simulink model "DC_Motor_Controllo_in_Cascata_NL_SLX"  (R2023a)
settings: Solver=ode45  StartTime=0.0  StopTime=10.0  MaxStep=0.001  RelTol=1e-3
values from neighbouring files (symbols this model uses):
  b_m = 0.002*N/(m/sec)    (= 0.002)    [DC_Motor_Controllo_in_Cascata_NL_SLX_m.m]    (also in DC_Motor_Controllo_in_Cascata_SLX_m.m; Electrical_DC_Motor_EQN.m; Electrical_DC_Motor_SLX_m.m)
  C_p_0 = 0*Nm    (= 0)    [DC_Motor_Controllo_in_Cascata_NL_SLX_m.m]    (also in DC_Motor_Controllo_in_Cascata_SLX_m.m; Electrical_DC_Motor_SLX_m.m)
  I_a_0 = 0*A    (= 0)    [DC_Motor_Controllo_in_Cascata_NL_SLX_m.m]    (also in DC_Motor_Controllo_in_Cascata_SLX_m.m; Electrical_DC_Motor_SLX_m.m)
  J_m = 0.01*kg*m^2    (= 0.01)    [DC_Motor_Controllo_in_Cascata_NL_SLX_m.m]    (also in DC_Motor_Controllo_in_Cascata_SLX_m.m; Electrical_DC_Motor_EQN.m; Electrical_DC_Motor_SLX_m.m)
  K_I1 = 12532    [DC_Motor_Controllo_in_Cascata_NL_SLX_m.m]    (also in DC_Motor_Controllo_in_Cascata_SLX_m.m)
  K_m = 0.5    [DC_Motor_Controllo_in_Cascata_NL_SLX_m.m]    (also in DC_Motor_Controllo_in_Cascata_SLX_m.m; Electrical_DC_Motor_EQN.m; Electrical_DC_Motor_SLX_m.m)
  K_Thm = 100    [DC_Motor_Controllo_in_Cascata_NL_SLX_m.m]    (also in DC_Motor_Controllo_in_Cascata_SLX_m.m)
  K_wm = 4    [DC_Motor_Controllo_in_Cascata_NL_SLX_m.m]    (also in DC_Motor_Controllo_in_Cascata_SLX_m.m)
  L_a = 0.003*H    (= 0.003)    [DC_Motor_Controllo_in_Cascata_NL_SLX_m.m]    (also in DC_Motor_Controllo_in_Cascata_SLX_m.m; Electrical_DC_Motor_EQN.m; Electrical_DC_Motor_SLX_m.m)
  Max_V1 = 500*V    (= 500)    [DC_Motor_Controllo_in_Cascata_NL_SLX_m.m]
  R_a = 1*Ohm    (= 1)    [DC_Motor_Controllo_in_Cascata_NL_SLX_m.m]    (also in DC_Motor_Controllo_in_Cascata_SLX_m.m; Electrical_DC_Motor_EQN.m; Electrical_DC_Motor_SLX_m.m)
  Th_ref = 100*giri    (= 628.318530718)    [DC_Motor_Controllo_in_Cascata_NL_SLX_m.m]    (also in DC_Motor_Controllo_in_Cascata_SLX_m.m)
  Thm_0 = 0    [DC_Motor_Controllo_in_Cascata_NL_SLX_m.m]    (also in DC_Motor_Controllo_in_Cascata_SLX_m.m)
  Ts = Tfin/Nr_Ts_Points    (= 0.00075)    [DC_Motor_Controllo_in_Cascata_NL_SLX_m.m]    (also in DC_Motor_Controllo_in_Cascata_SLX_m.m = 5e-05; Electrical_DC_Motor_SLX_m.m = 0.000163975)
  w_m_0 = 0*rad/sec    (= 0)    [DC_Motor_Controllo_in_Cascata_NL_SLX_m.m]    (also in DC_Motor_Controllo_in_Cascata_SLX_m.m; Electrical_DC_Motor_SLX_m.m)

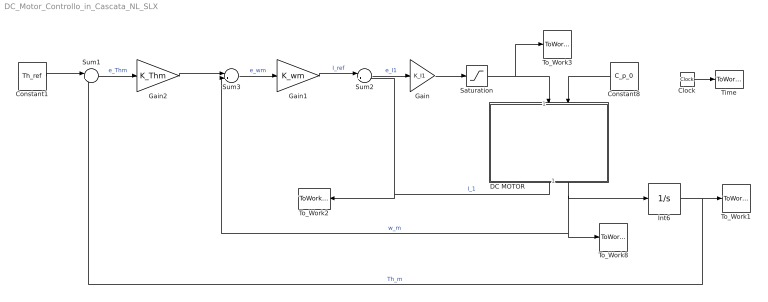
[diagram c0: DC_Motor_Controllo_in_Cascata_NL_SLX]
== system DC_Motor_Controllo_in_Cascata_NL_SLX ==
  Clock : Clock
  Constant1 : Constant  Value=Th_ref
  Constant8 : Constant  Value=C_p_0
  DC MOTOR : Subsystem
  Gain : Gain  Gain=K_I1
  Gain1 : Gain  Gain=K_wm
  Gain2 : Gain  Gain=K_Thm
  Int6 : Integrator  InitialCondition=Thm_0
  Saturation : Saturate  UpperLimit=Max_V1  LowerLimit=-Max_V1  ZeroCross=off
  Sum1 : Sum  Inputs=|+-
  Sum2 : Sum  Inputs=|+-
  Sum3 : Sum  Inputs=|+-
  Time : ToWorkspace  VariableName=t  SaveFormat=Timeseries  SampleTime=Ts
  To_Work1 : ToWorkspace  VariableName=Th_m  SaveFormat=Timeseries  SampleTime=Ts
  To_Work2 : ToWorkspace  VariableName=I_1  SaveFormat=Timeseries  SampleTime=Ts
  To_Work3 : ToWorkspace  VariableName=V_1  SaveFormat=Timeseries  SampleTime=Ts
  To_Work8 : ToWorkspace  VariableName=w_m  SaveFormat=Timeseries  SampleTime=Ts
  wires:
  Clock/1 -> Time/1
  Constant8/1 -> DC MOTOR/2(In2)
  DC MOTOR/2(w_m) -> To_Work8/1, Sum3/2, Int6/1  "w_m"
  DC MOTOR/1(I_1) -> Sum2/2, To_Work2/1  "I_1"
  Sum2/1 -> Gain/1  "e_I1"
  Gain/1 -> Saturation/1
  Int6/1 -> Sum1/2, To_Work1/1  "Th_m"
  Sum3/1 -> Gain1/1  "e_wm"
  Gain1/1 -> Sum2/1  "I_ref"
  Sum1/1 -> Gain2/1  "e_Thm"
  Constant1/1 -> Sum1/1
  Gain2/1 -> Sum3/1
  Saturation/1 -> DC MOTOR/1(In1), To_Work3/1

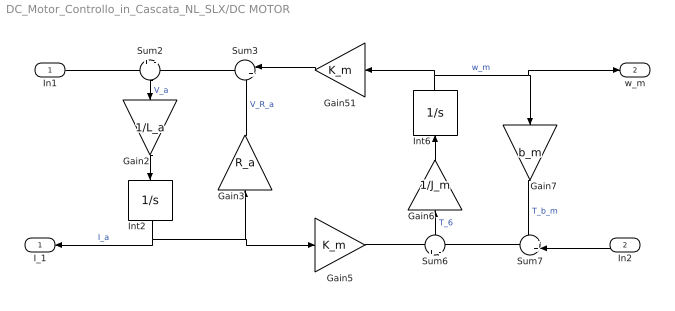
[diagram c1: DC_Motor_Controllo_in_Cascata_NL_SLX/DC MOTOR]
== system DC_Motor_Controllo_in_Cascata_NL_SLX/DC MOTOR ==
  In1 : Inport
  In2 : Inport  Port=2
  Gain2 : Gain  Gain=1/L_a  Multiplication=Matrix(K*u)
  Gain3 : Gain  Gain=R_a  Multiplication=Matrix(K*u)
  Gain5 : Gain  Gain=K_m  Multiplication=Matrix(K*u)
  Gain51 : Gain  Gain=K_m  Multiplication=Matrix(K*u)
  Gain6 : Gain  Gain=1/J_m  Multiplication=Matrix(K*u)
  Gain7 : Gain  Gain=b_m  Multiplication=Matrix(K*u)
  Int2 : Integrator  InitialCondition=I_a_0
  Int6 : Integrator  InitialCondition=w_m_0
  Sum2 : Sum  Inputs=+|-
  Sum3 : Sum  Inputs=|++
  Sum6 : Sum  Inputs=+|-
  Sum7 : Sum  Inputs=++|
  I_1 : Outport
  w_m : Outport  Port=2
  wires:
  Gain6/1 -> Int6/1
  Gain5/1 -> Sum6/1
  Int2/1 -> I_1/1, Gain3/1, Gain5/1  "I_a"
  Sum7/1 -> Sum6/2
  Int6/1 -> Gain51/1, w_m/1, Gain7/1  "w_m"
  Gain51/1 -> Sum3/1
  Gain2/1 -> Int2/1
  Gain3/1 -> Sum3/2  "V_R_a"
  Sum3/1 -> Sum2/2
  Sum6/1 -> Gain6/1  "T_6"
  Sum2/1 -> Gain2/1  "V_a"
  Gain7/1 -> Sum7/1  "T_b_m"
  In2/1 -> Sum7/2
  In1/1 -> Sum2/1
